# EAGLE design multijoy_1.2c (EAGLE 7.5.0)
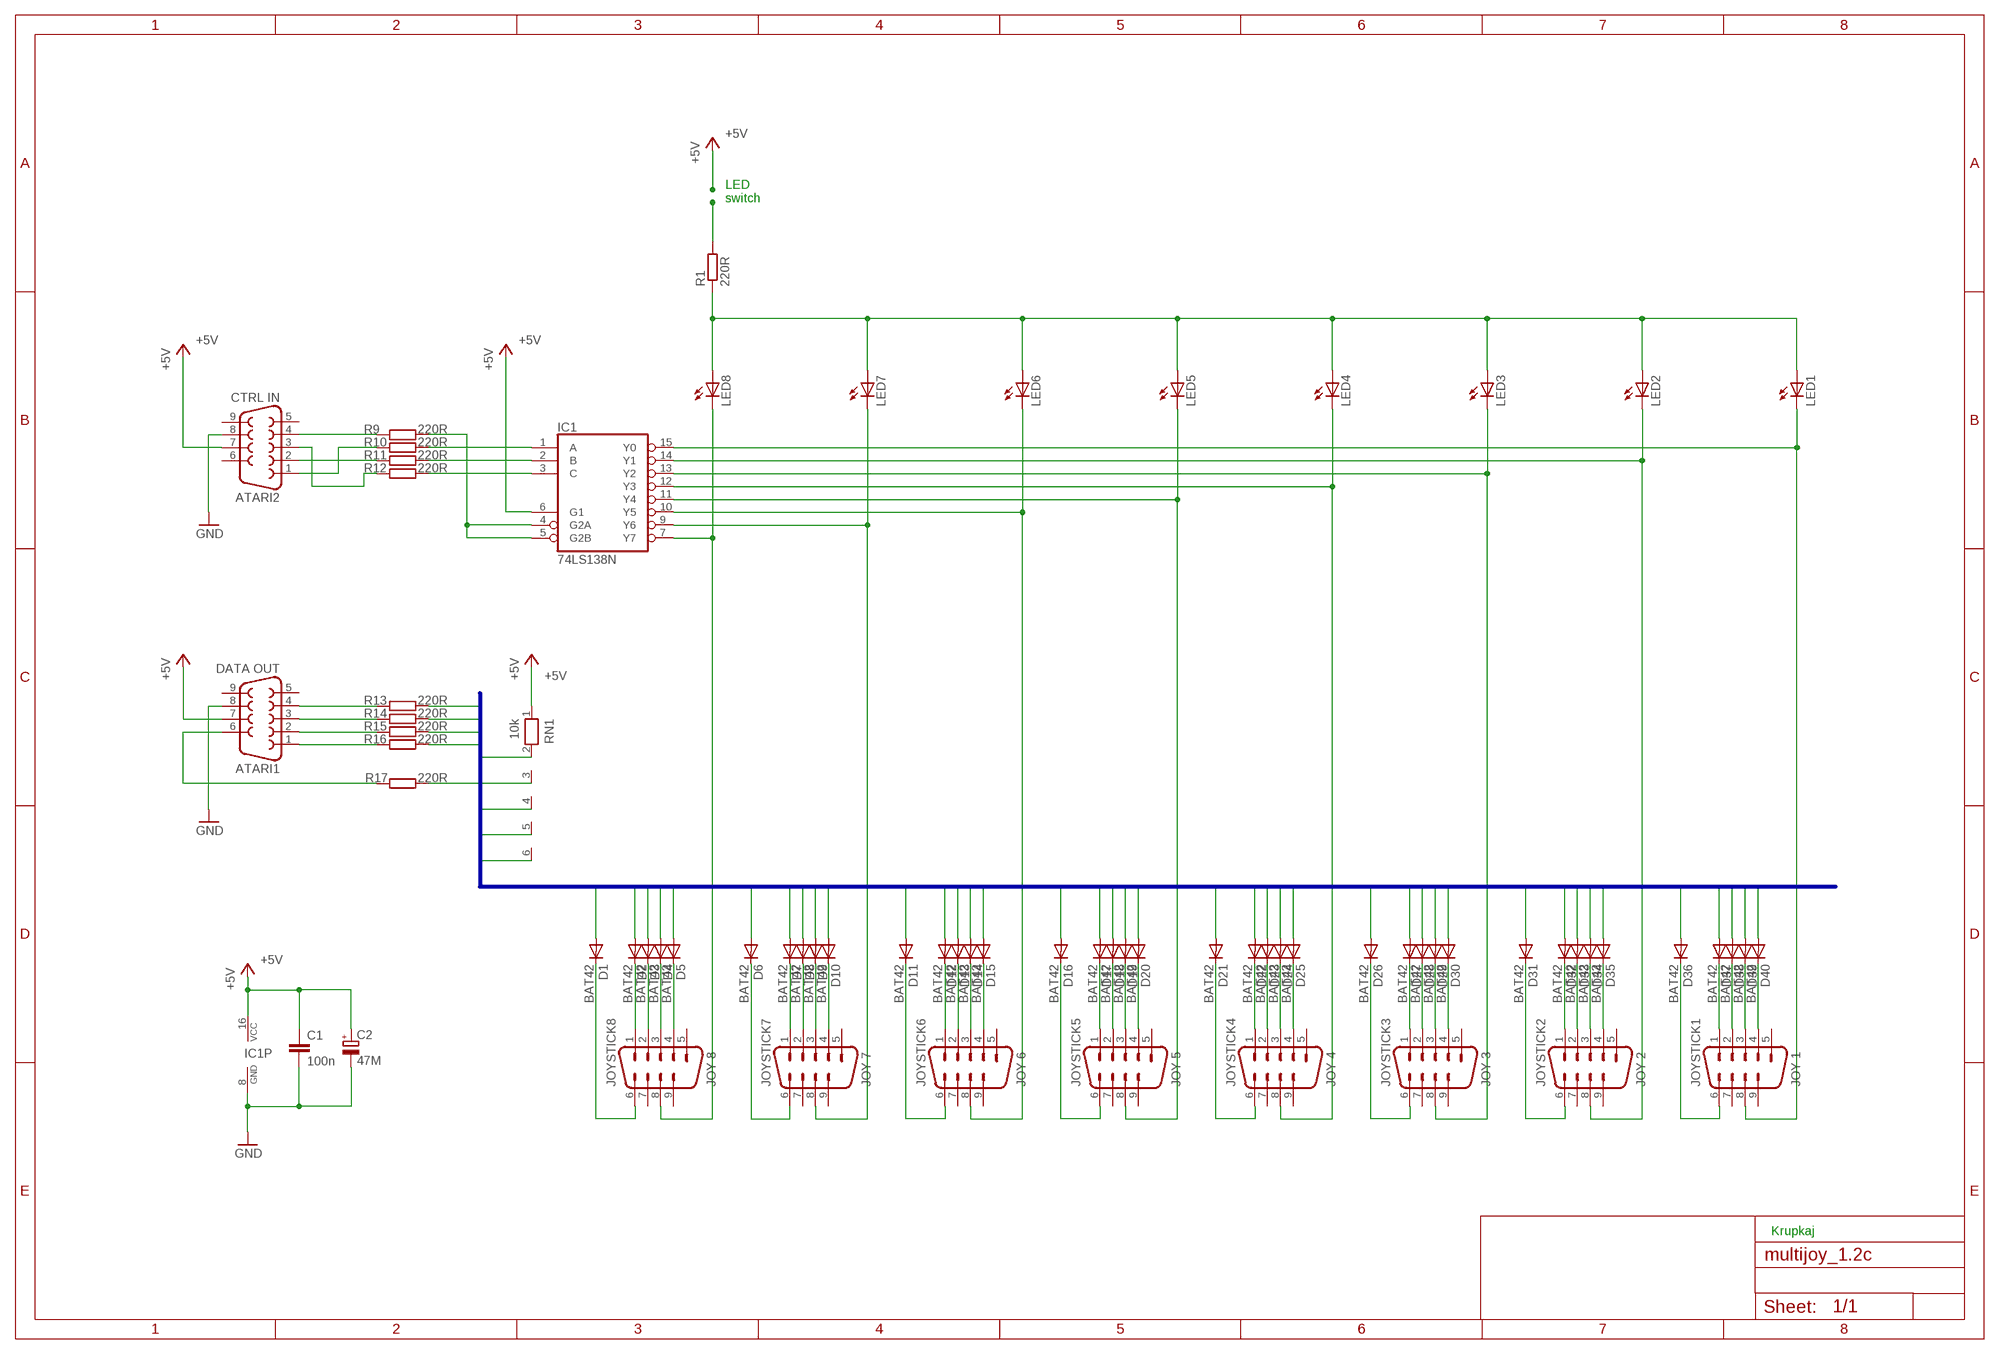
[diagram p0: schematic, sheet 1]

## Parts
ATARI1  DATA OUT  F09HP  [F09HP]
ATARI2  CTRL IN  F09HP  [F09HP]
C1  100n  C-EU050-025X075  [C050-025X075]
C2  47M  CPOL-EUE2,5-6E  [E2,5-6E]
D1  BAT42  DIODE-D-5  [D-5]
D2  BAT42  1N4148D-5  [D-5]
D3  BAT42  DIODE-D-7.5  [D-7.5]
D4  BAT42  DIODE-D-10  [D-10]
D5  BAT42  1N4148D-12.5  [D-12.5]
D6  BAT42  1N4148D-7.5  [D-7.5]
D7  BAT42  1N4148D-5  [D-5]
D8  BAT42  DIODE-D-10  [D-10]
D9  BAT42  DIODE-D-10  [D-10]
D10  BAT42  1N4148D-12.5  [D-12.5]
D11  BAT42  1N4148D-7.5  [D-7.5]
D12  BAT42  1N4148D-5  [D-5]
D13  BAT42  1N4148D-10  [D-10]
D14  BAT42  1N4148D-10  [D-10]
D15  BAT42  1N4148D-12.5  [D-12.5]
D16  BAT42  1N4148D-5  [D-5]
D17  BAT42  1N4148D-7.5  [D-7.5]
D18  BAT42  1N4148D-7.5  [D-7.5]
D19  BAT42  1N4148D-10  [D-10]
D20  BAT42  1N4148D-12.5  [D-12.5]
D21  BAT42  1N4148D-7.5  [D-7.5]
D22  BAT42  1N4148D-5  [D-5]
D23  BAT42  1N4148D-7.5  [D-7.5]
D24  BAT42  1N4148D-10  [D-10]
D25  BAT42  1N4148D-12.5  [D-12.5]
D26  BAT42  1N4148D-7.5  [D-7.5]
D27  BAT42  1N4148D-7.5  [D-7.5]
D28  BAT42  1N4148D-10  [D-10]
D29  BAT42  1N4148D-10  [D-10]
D30  BAT42  1N4148D-12.5  [D-12.5]
D31  BAT42  1N4148D-7.5  [D-7.5]
D32  BAT42  1N4148D-5  [D-5]
D33  BAT42  1N4148D-10  [D-10]
D34  BAT42  1N4148D-10  [D-10]
D35  BAT42  1N4148D-12.5  [D-12.5]
D36  BAT42  1N4148D-7.5  [D-7.5]
D37  BAT42  1N4148D-7.5  [D-7.5]
D38  BAT42  1N4148D-7.5  [D-7.5]
D39  BAT42  1N4148D-7.5  [D-7.5]
D40  BAT42  1N4148D-7.5  [D-7.5]
IC1  74LS138N  [DIL16]
JOYSTICK1  JOY 1  M09HP  [M09HP]
JOYSTICK2  JOY 2  M09HP  [M09HP]
JOYSTICK3  JOY 3  M09HP  [M09HP]
JOYSTICK4  JOY 4  M09HP  [M09HP]
JOYSTICK5  JOY 5  M09HP  [M09HP]
JOYSTICK6  JOY 6  M09HP  [M09HP]
JOYSTICK7  JOY 7  M09HP  [M09HP]
JOYSTICK8  JOY 8  M09HP  [M09HP]
LED1  LEDCHIPLED_0805  [CHIPLED_0805]
LED2  LEDCHIPLED_0805  [CHIPLED_0805]
LED3  LEDCHIPLED_0805  [CHIPLED_0805]
LED4  LEDCHIPLED_0805  [CHIPLED_0805]
LED5  LEDCHIPLED_0805  [CHIPLED_0805]
LED6  LEDCHIPLED_0805  [CHIPLED_0805]
LED7  LEDCHIPLED_0805  [CHIPLED_0805]
LED8  LEDCHIPLED_0805  [CHIPLED_0805]
R1  220R  R-EU_R0805  [R0805]
R9  220R  R-EU_R0805  [R0805]
R10  220R  R-EU_R0805  [R0805]
R11  220R  R-EU_R0805  [R0805]
R12  220R  R-EU_R0805  [R0805]
R13  220R  R-EU_R0805  [R0805]
R14  220R  R-EU_R0805  [R0805]
R15  220R  R-EU_R0805  [R0805]
R16  220R  R-EU_R0805  [R0805]
R17  220R  R-EU_R0805  [R0805]
RN1  10k  RN05  [RN-6]

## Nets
+5V: ATARI1.7 ATARI2.7 C1.1 C2.+ IC1.6(G1) IC1.16(VCC) RN1.1
+5VLED: R1.2
GND: ATARI1.8 ATARI2.8 C1.2 C2.- IC1.8(GND)
INPUT1: D2.A D7.A D12.A D17.A D22.A D27.A D32.A D37.A R16.2 RN1.6
INPUT2: D3.A D8.A D13.A D18.A D23.A D28.A D33.A D38.A R15.2 RN1.4
INPUT3: D4.A D9.A D14.A D19.A D24.A D29.A D34.A D39.A R14.2 RN1.3
INPUT4: D5.A D10.A D15.A D20.A D25.A D30.A D35.A D40.A R13.2 RN1.2
INPUT6: D1.A D6.A D11.A D16.A D21.A D26.A D31.A D36.A R17.2 RN1.5
N$1: D39.C JOYSTICK1.3
N$2: D40.C JOYSTICK1.4
N$3: D38.C JOYSTICK1.2
N$4: D37.C JOYSTICK1.1
N$5: D1.C JOYSTICK8.6
N$6: D2.C JOYSTICK8.1
N$7: D3.C JOYSTICK8.2
N$8: D4.C JOYSTICK8.3
N$9: D5.C JOYSTICK8.4
N$10: D6.C JOYSTICK7.6
N$11: D7.C JOYSTICK7.1
N$12: D8.C JOYSTICK7.2
N$13: D9.C JOYSTICK7.3
N$14: D10.C JOYSTICK7.4
N$15: D36.C JOYSTICK1.6
N$16: D35.C JOYSTICK2.4
N$17: D34.C JOYSTICK2.3
N$18: D33.C JOYSTICK2.2
N$19: D32.C JOYSTICK2.1
N$20: D31.C JOYSTICK2.6
N$21: D30.C JOYSTICK3.4
N$22: D27.C JOYSTICK3.1
N$23: D26.C JOYSTICK3.6
N$24: D25.C JOYSTICK4.4
N$25: D24.C JOYSTICK4.3
N$26: D23.C JOYSTICK4.2
N$27: D22.C JOYSTICK4.1
N$28: D21.C JOYSTICK4.6
N$29: D20.C JOYSTICK5.4
N$30: D19.C JOYSTICK5.3
N$31: D18.C JOYSTICK5.2
N$32: D17.C JOYSTICK5.1
N$33: D16.C JOYSTICK5.6
N$34: D15.C JOYSTICK6.4
N$35: D14.C JOYSTICK6.3
N$36: D13.C JOYSTICK6.2
N$37: D12.C JOYSTICK6.1
N$38: D11.C JOYSTICK6.6
N$39: D28.C JOYSTICK3.2
N$40: D29.C JOYSTICK3.3
N$41: IC1.7(Y7) JOYSTICK8.8 LED8.C
N$43: IC1.10(Y5) JOYSTICK6.8 LED6.C
N$44: IC1.11(Y4) JOYSTICK5.8 LED5.C
N$45: IC1.12(Y3) JOYSTICK4.8 LED4.C
N$46: IC1.13(Y2) JOYSTICK3.8 LED3.C
N$47: IC1.14(Y1) JOYSTICK2.8 LED2.C
N$48: IC1.15(Y0) JOYSTICK1.8 LED1.C
N$49: IC1.1(A) R10.2
N$51: ATARI2.3 R12.1
N$52: IC1.4(G2A) IC1.5(G2B) R9.2
N$67: LED1.A LED2.A LED3.A LED4.A LED5.A LED6.A LED7.A LED8.A R1.1
N$68: ATARI2.4 R9.1
N$69: ATARI2.1 R10.1
N$70: ATARI2.2 R11.1
N$71: IC1.3(C) R12.2
N$73: ATARI1.4 R13.1
N$74: ATARI1.3 R14.1
N$75: ATARI1.2 R15.1
N$76: ATARI1.1 R16.1
N$77: ATARI1.6 R17.1
N$724: IC1.9(Y6) JOYSTICK7.8 LED7.C
OUTPUT: IC1.2(B) R11.2
Unconnected: ATARI1.5 ATARI1.9 ATARI2.5 ATARI2.6 ATARI2.9 JOYSTICK1.5 JOYSTICK1.7 JOYSTICK1.9 JOYSTICK2.5 JOYSTICK2.7 JOYSTICK2.9 JOYSTICK3.5 JOYSTICK3.7 JOYSTICK3.9 JOYSTICK4.5 JOYSTICK4.7 JOYSTICK4.9 JOYSTICK5.5 JOYSTICK5.7 JOYSTICK5.9 JOYSTICK6.5 JOYSTICK6.7 JOYSTICK6.9 JOYSTICK7.5 JOYSTICK7.7 JOYSTICK7.9 JOYSTICK8.5 JOYSTICK8.7 JOYSTICK8.9

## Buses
INPUT[1..6]

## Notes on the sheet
- LED
  switch
- Krupkaj

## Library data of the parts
ATARI1 ATARI2 = con-subd-m:F09: SUB-D; OC_FARNELL: unknown; OC_NEWARK: unknown
C1 = rcl:C-EU: CAPACITOR, European symbol
C2 = rcl:CPOL-EU: POLARIZED CAPACITOR, European symbol
D1 D3 D4 D8 D9 = diode:DIODE-: DIODE
D2 D5-D7 D10-D40 = diode:1N4148: DIODE
IC1 = 74xx-eu:74*138: 3-line to 8-line DECODER/DEMULTIPLEXER
JOYSTICK1-JOYSTICK8 = con-subd-m:M09: SUB-D; OC_FARNELL: unknown; OC_NEWARK: unknown
LED1-LED8 = led:LED: LED
R1 R9-R17 = rcl:R-EU_: RESISTOR, European symbol
RN1 = resistor-net:RN05: RESISTOR NETWORK

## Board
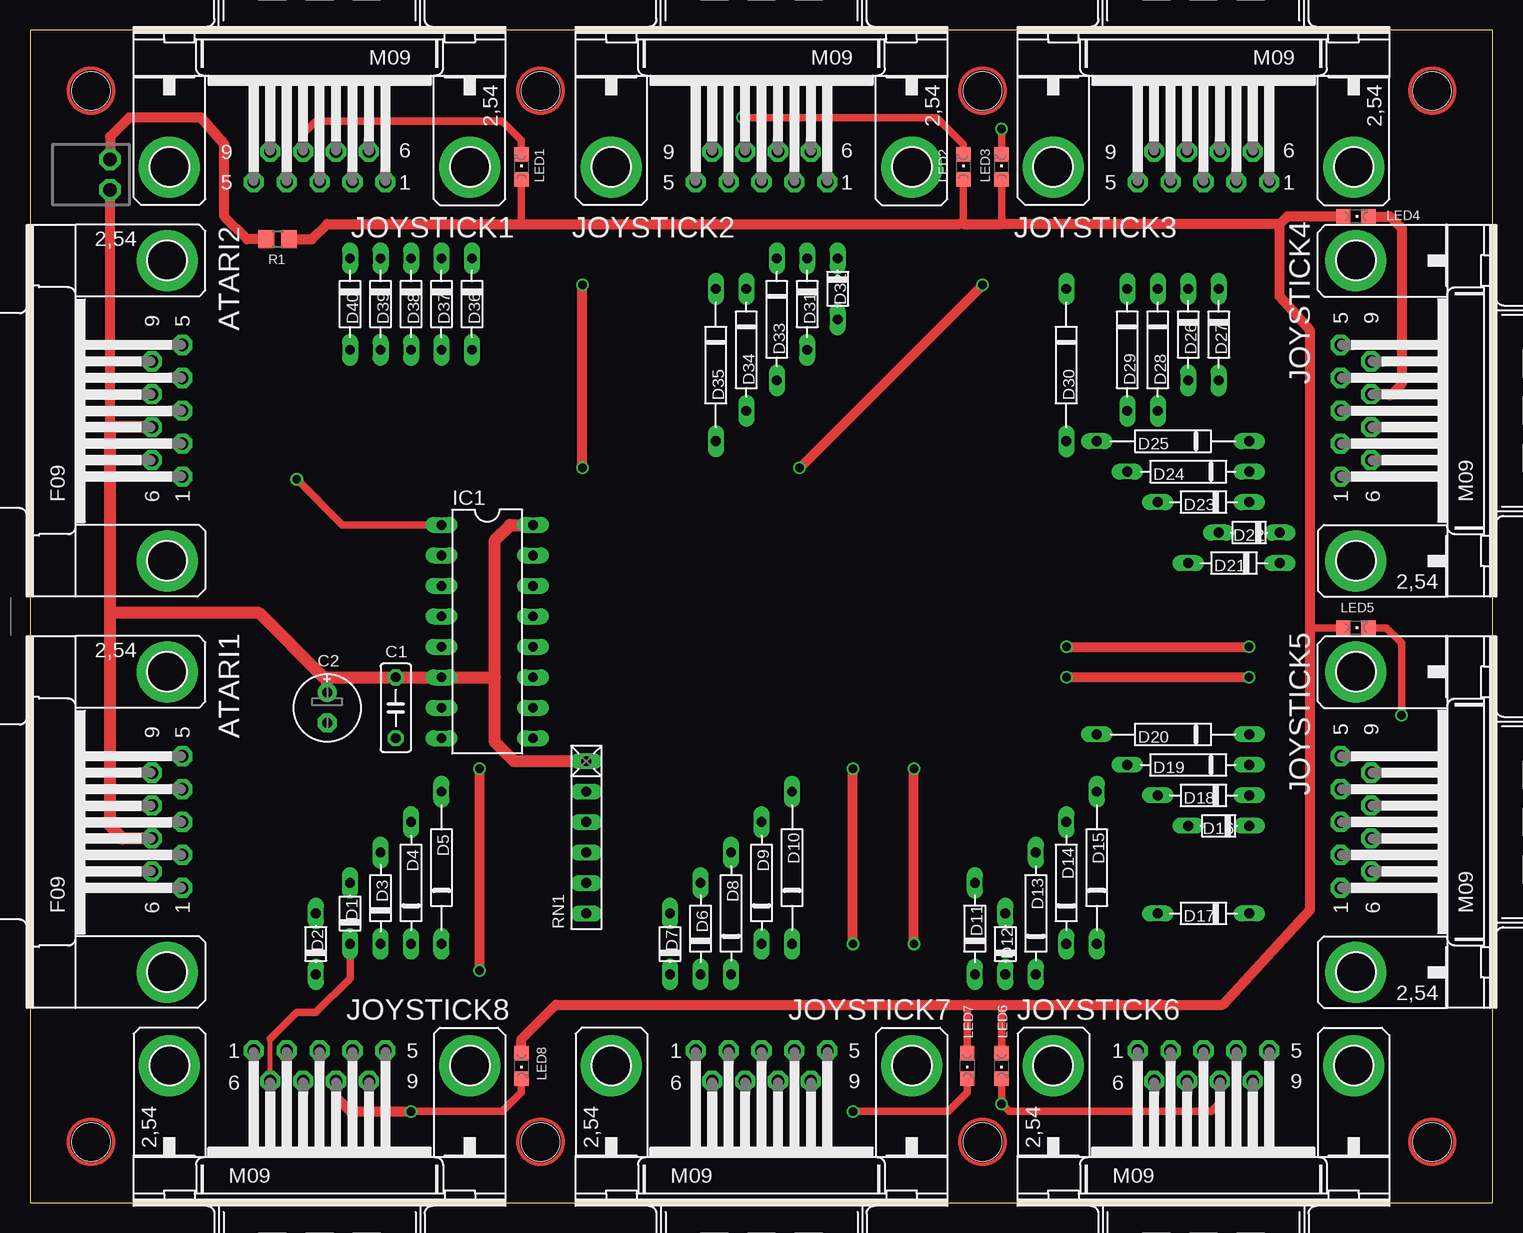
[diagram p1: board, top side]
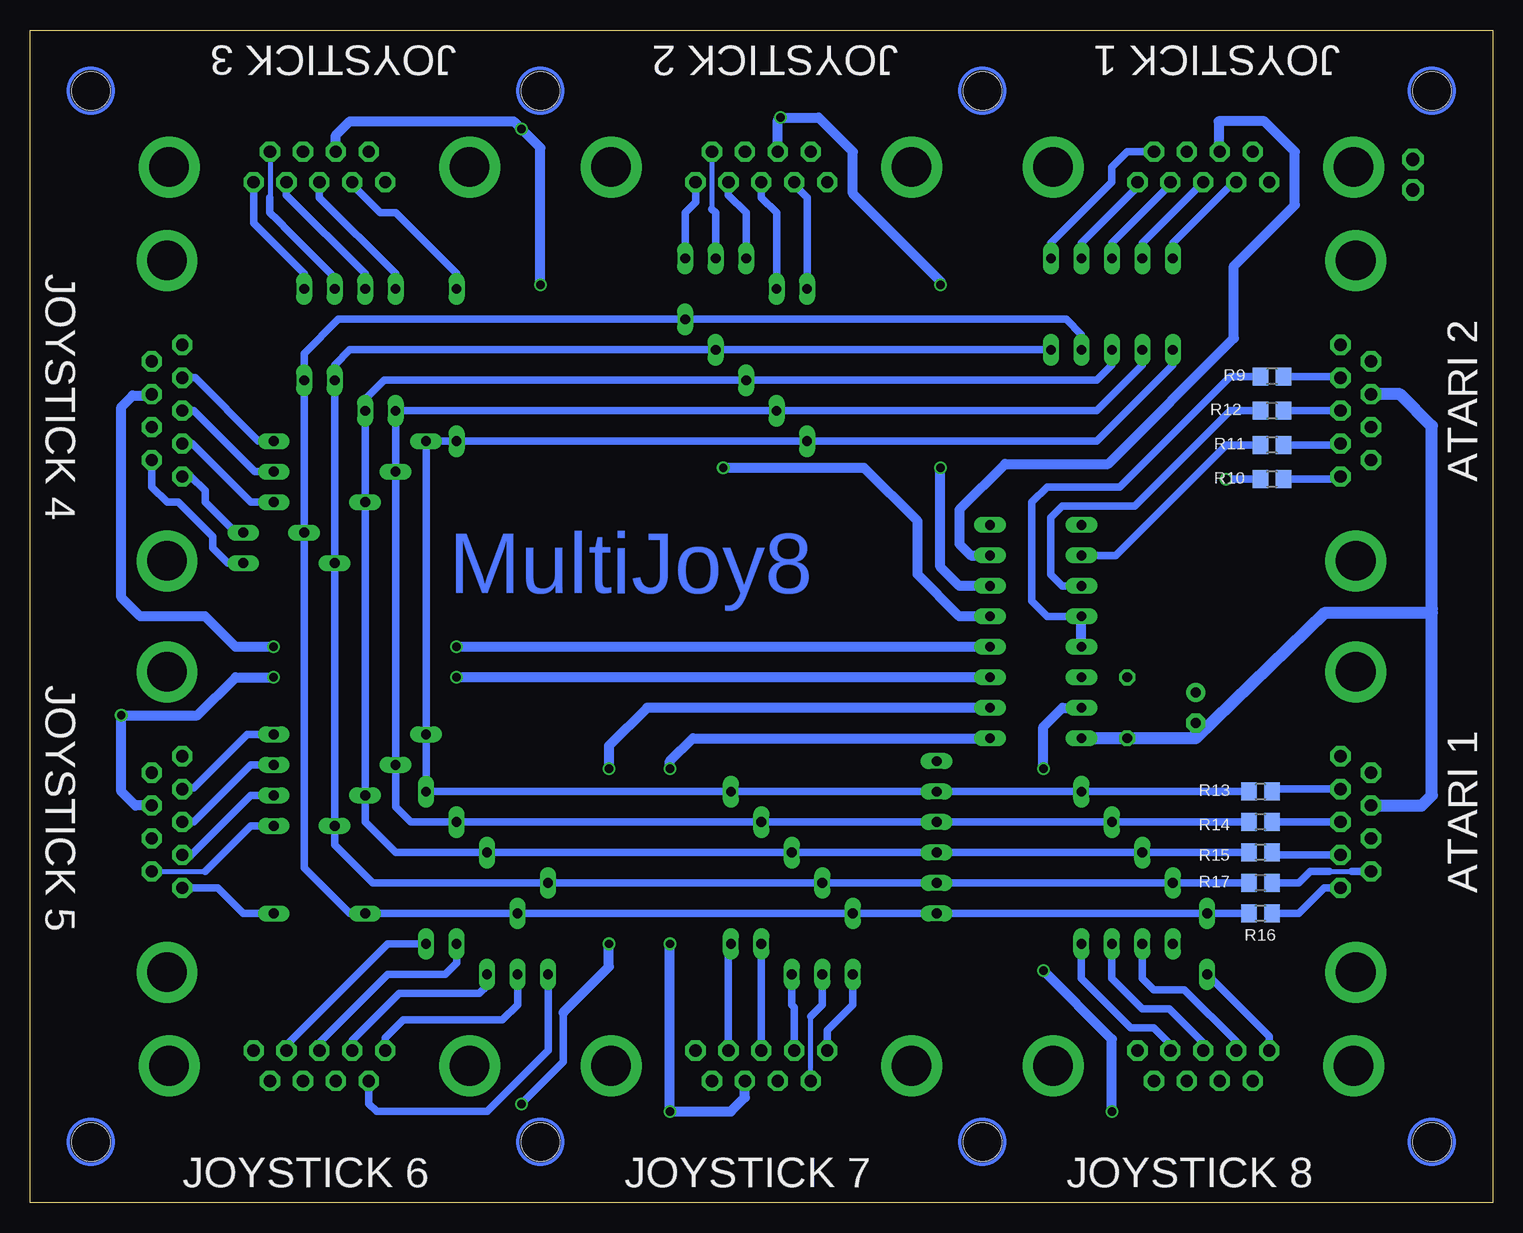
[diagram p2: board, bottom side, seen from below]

Size 121.91 x 97.78 mm. Coordinates in mm from the lower left corner, seen from the top.
Outline: 0,0 121.91,0 121.91,97.78 0,97.78 0,0
Copper layers (1*16): Top 0.035mm / dielectric 1.5mm / Bottom 0.035mm
Design rules "SeeedStudio_2layer_DRU_no_angle_20140221": minimum track width 6mil, minimum drill 12mil, track to track 6mil, track to pad 6mil, pad to pad 6mil, via to via 6mil, smd to smd 0mil, copper to edge 10mil, drill to drill 10mil, minimum pad ring 10mil, minimum via ring 6mil, stop-mask expansion 2mil, vias tented up to drill 100mil, thermal gap 10mil
Holes 3.2 mm at 5.08,92.71 42.55,92.71 79.38,92.71 116.84,92.71 116.84,5.08 79.38,5.08 42.55,5.08 5.08,5.08

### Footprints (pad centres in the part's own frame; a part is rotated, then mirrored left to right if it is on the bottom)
F09HP = drill 1.016 pad 1.676 octagon: 1 -5.486,-1.27; 2 -2.743,-1.27; 3 0,-1.27; 4 2.743,-1.27; 5 5.486,-1.27; 6 -4.115,1.27; 7 -1.372,1.27; 8 1.372,1.27; 9 4.115,1.27 | drill 3.302 pad 5.08: G1 -12.522,0; G2 12.522,0
C050-025X075 = drill 0.813 octagon: 1 -2.54,0; 2 2.54,0
E2,5-6E = drill 0.813 pad 1.575: + -1.27,0 | drill 0.813 pad 1.575 octagon: - 1.27,0
D-5 = drill 0.813 long: A 2.54,0; C -2.54,0
D-7.5 = drill 0.813 long: A 3.81,0; C -3.81,0
D-10 = drill 0.813 long: A 5.08,0; C -5.08,0
D-12.5 = drill 0.813 long: A 6.35,0; C -6.35,0
DIL16 = drill 0.813 long: 1 -8.89,-3.81; 2 -6.35,-3.81; 3 -3.81,-3.81; 4 -1.27,-3.81; 5 1.27,-3.81; 6 3.81,-3.81; 7 6.35,-3.81; 8 8.89,-3.81; 9 8.89,3.81; 10 6.35,3.81; 11 3.81,3.81; 12 1.27,3.81; 13 -1.27,3.81; 14 -3.81,3.81; 15 -6.35,3.81; 16 -8.89,3.81
M09HP = drill 1.016 pad 1.676 octagon: 1 -5.486,1.27; 2 -2.743,1.27; 3 0,1.27; 4 2.743,1.27; 5 5.486,1.27; 6 -4.115,-1.27; 7 -1.372,-1.27; 8 1.372,-1.27; 9 4.115,-1.27 | drill 3.302 pad 5.08: G1 -12.522,0; G2 12.522,0
CHIPLED_0805 = smd 1.2 x 1.2: A 0,-1.05; C 0,1.05
R0805 = smd 1.3 x 1.5: 1 -0.95,0; 2 0.95,0
RN-6 = drill 0.813 long: 1 -6.35,0; 2 -3.81,0; 3 -1.27,0; 4 1.27,0; 5 3.81,0; 6 6.35,0

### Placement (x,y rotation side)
ATARI1  11.43,31.75 90 top
ATARI2  11.43,66.04 90 top
C1  30.48,41.27 270 top
C2  24.77,41.27 270 top
D1  26.67,24.13 90 top
D2  23.81,21.59 90 top
D3  29.21,25.4 90 top
D4  31.75,26.67 90 top
D5  34.29,27.94 90 top
D6  55.88,22.86 90 top
D7  53.34,21.59 90 top
D8  58.42,24.13 90 top
D9  60.96,26.67 90 top
D10  63.5,27.94 90 top
D11  78.74,22.86 90 top
D12  81.28,21.59 90 top
D13  83.82,24.13 90 top
D14  86.36,26.67 90 top
D15  88.9,27.94 90 top
D16  99.06,31.43 180 top
D17  97.79,24.13 180 top
D18  97.79,33.97 180 top
D19  96.52,36.51 180 top
D20  95.25,39.05 180 top
D21  100.33,53.34 180 top
D22  101.6,55.88 180 top
D23  97.79,58.42 180 top
D24  96.52,60.96 180 top
D25  95.25,63.5 180 top
D26  96.52,72.39 270 top
D27  99.06,72.39 270 top
D28  93.98,71.12 270 top
D29  91.44,71.12 270 top
D30  86.36,69.85 270 top
D31  64.77,74.93 270 top
D32  67.31,76.2 270 top
D33  62.23,73.66 270 top
D34  59.69,71.12 270 top
D35  57.15,69.85 270 top
D36  36.83,74.93 270 top
D37  34.29,74.93 270 top
D38  31.75,74.93 270 top
D39  29.21,74.93 270 top
D40  26.67,74.93 270 top
IC1  38.1,47.62 270 top
JOYSTICK1  24.13,86.36 180 top
JOYSTICK2  60.96,86.36 180 top
JOYSTICK3  97.79,86.36 180 top
JOYSTICK4  110.49,66.04 90 top
JOYSTICK5  110.49,31.75 90 top
JOYSTICK6  97.79,11.43 0 top
JOYSTICK7  60.96,11.43 0 top
JOYSTICK8  24.13,11.43 0 top
LED1  40.96,86.36 0 top
LED2  77.79,86.36 0 top
LED3  80.96,86.36 0 top
LED4  110.49,82.23 270 top
LED5  110.49,47.94 270 top
LED6  80.96,11.43 180 top
LED7  78.1,11.43 180 top
LED8  40.96,11.43 180 top
R1  20.64,80.33 180 top
R9  18.41,68.9 180 bottom
R10  18.41,60.33 180 bottom
R11  18.41,63.18 180 bottom
R12  18.41,66.04 180 bottom
R13  19.37,34.29 180 bottom
R14  19.37,31.75 180 bottom
R15  19.37,29.21 180 bottom
R16  19.37,24.13 180 bottom
R17  19.37,26.67 180 bottom
RN1  46.36,30.48 270 top

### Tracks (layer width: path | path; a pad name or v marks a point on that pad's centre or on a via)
+5V  (via drill 1.1 pad 1.78)
  Top 0.813: 6.67,64.67 v6.67,84.45 | 6.67,31.75 6.67,31.43
  Top 1.016: IC1.16 40,56.52 38.73,55.25 38.73,43.81 | 38.73,43.81 IC1.6 C1.1 24.77,43.81 | 6.67,49.21 19.05,49.21 24.45,43.81 24.77,43.81 | 38.73,43.81 38.73,38.42 40.32,36.83 RN1.1 | C2.+ 24.77,43.81 | ATARI2.7 6.67,64.67 6.67,49.21 | ATARI1.7 7.72,30.38 6.67,31.43 | 6.67,31.75 6.67,49.21
+5VLED  (via drill 1.1 pad 1.78)
  Top 0.813: R1.2 18.1,80.33 16.19,82.23 16.19,88.27 14.29,90.49 8.26,90.49 6.67,88.9 v6.67,86.99
GND
  Bottom 1.016: 24.77,38.73 13.97,49.21 5.08,49.21 | 5.08,49.21 5.08,49.53 5.08,64.77 7.72,67.41 ATARI2.8 | 24.77,38.73 C1.2 IC1.8 | C2.- 24.77,38.73 | ATARI1.8 5.93,33.12 5.08,33.97 5.08,49.21
INPUT1
  Bottom 0.61: D37.A 34.29,72.39 35.56,73.66 D32.A 96.2,73.66 99.06,70.8 D27.A D22.A 99.06,27.94 95.25,24.13 D17.A D12.A D7.A RN1.6 D2.A R16.2
INPUT2
  Bottom 0.61: D38.A 31.75,69.85 33.02,68.58 D33.A 92.39,68.58 93.98,66.99 D28.A D23.A D18.A 93.98,31.75 91.44,29.21 D13.A D8.A RN1.4 D3.A R15.2
INPUT3
  Bottom 0.61: D39.A 29.21,69.85 33.02,66.04 D34.A D29.A D24.A D19.A 91.44,33.02 90.17,31.75 D14.A D9.A RN1.3 D4.A R14.2
INPUT4
  Bottom 0.61: D40.A 26.67,69.85 33.02,63.5 D35.A D30.A D25.A D20.A D15.A D10.A RN1.2 D5.A R13.2
INPUT6
  Bottom 0.61: D36.A D31.A 95.25,71.12 96.52,69.85 D26.A D21.A D16.A 96.52,29.84 93.34,26.67 D11.A D6.A RN1.5 D1.A R17.2
N$1
  Bottom 0.406: 29.21,80.01 D39.C
  Bottom 0.61: JOYSTICK1.3 29.21,80.01
N$2
  Bottom 0.406: JOYSTICK1.4 21.39,85.29 | 26.67,80.01 D40.C
  Bottom 0.61: 21.39,85.29 26.67,80.01
N$3
  Bottom 0.406: JOYSTICK1.2 26.87,84.89 | 31.75,80.01 D38.C
  Bottom 0.61: 26.87,84.89 31.75,80.01
N$4
  Bottom 0.406: JOYSTICK1.1 29.62,84.68 | 34.29,80.01 D37.C
  Bottom 0.61: 29.62,84.68 34.29,80.01
N$5
  Top 0.406: JOYSTICK8.6 20.02,13.66
  Top 0.61: 20.02,13.66 22.23,15.88 23.81,15.88 26.67,18.73 D1.C
N$6
  Bottom 0.61: JOYSTICK8.1 18.64,13.88 D2.C
N$7
  Bottom 0.61: JOYSTICK8.2 21.39,13.45 25.72,17.78 28.26,17.78 29.21,18.73 D3.C
N$8
  Bottom 0.61: JOYSTICK8.3 24.13,13.34 26.99,16.19 29.21,16.19 31.75,18.73 D4.C
N$9
  Bottom 0.61: JOYSTICK8.4 26.87,13.22 28.26,14.61 30.16,14.61 34.29,18.73 D5.C
N$10
  Bottom 0.406: JOYSTICK7.6 56.84,15.54
  Bottom 0.61: 56.84,15.54 55.88,16.51 D6.C
N$11
  Bottom 0.61: JOYSTICK7.1 55.47,14.38 53.34,16.51 D7.C
N$12
  Bottom 0.61: JOYSTICK7.2 58.22,16.31 58.42,16.51 D8.C
N$13
  Bottom 0.61: D9.C JOYSTICK7.3
N$14
  Bottom 0.61: JOYSTICK7.4 63.7,21.39 D10.C
N$15
  Bottom 0.406: 36.83,80.01 D36.C
  Bottom 0.61: JOYSTICK1.6 30.48,87.63 31.75,86.36 31.75,85.09 36.83,80.01
N$16
  Bottom 0.406: JOYSTICK2.4 58.22,84.89
  Bottom 0.61: 58.22,84.89 57.15,83.82 D35.C
N$17
  Bottom 0.61: JOYSTICK2.3 60.96,83.82 59.69,82.55 D34.C
N$18
  Bottom 0.61: JOYSTICK2.2 63.7,84.02 62.23,82.55 D33.C
N$19
  Bottom 0.61: JOYSTICK2.1 66.45,83.41 67.31,82.55 D32.C
N$20
  Bottom 0.406: JOYSTICK2.6 65.08,82.85
  Bottom 0.61: 65.08,82.85 64.77,82.55 D31.C
N$21
  Bottom 0.61: D30.C 86.36,77.47 91.44,82.55 92.71,82.55 95.05,84.89 JOYSTICK3.4
N$22
  Bottom 0.61: D27.C 99.06,77.47 103.28,81.69 JOYSTICK3.1
N$23
  Bottom 0.406: JOYSTICK3.6 101.91,83.83 101.92,83.82
  Bottom 0.61: D26.C 96.52,77.15 100.33,80.96 101.28,81.91 101.92,82.55 101.92,83.82
N$24
  Bottom 0.61: JOYSTICK4.4 108.15,68.78 102.87,63.5 D25.C
N$25
  Bottom 0.61: D24.C 103.19,60.96 108.27,66.04 JOYSTICK4.3
N$26
  Bottom 0.61: D23.C 103.5,58.42 108.38,63.3 JOYSTICK4.2
N$27
  Bottom 0.61: 109.22,60.96 JOYSTICK4.1 108.5,60.55 107.31,59.37 107.31,58.42 105.09,56.2 104.77,55.88 D22.C
N$28
  Bottom 0.61: JOYSTICK4.6 111.76,59.69 110.49,58.42 109.54,58.42 106.68,55.56 106.68,54.61 105.41,53.34 D21.C
N$29
  Bottom 0.406: 109.11,34.61 JOYSTICK5.4
  Bottom 0.61: D20.C 103.82,39.05 108.27,34.61 109.11,34.61
N$30
  Bottom 0.61: D19.C 103.5,36.51 108.27,31.75 JOYSTICK5.3
N$31
  Bottom 0.406: 109.11,28.89 JOYSTICK5.2
  Bottom 0.61: D18.C 103.5,33.97 108.58,28.89 109.11,28.89
N$32
  Bottom 0.61: D17.C 104.14,24.13 106.27,26.26 JOYSTICK5.1
N$33
  Bottom 0.406: JOYSTICK5.6 107.3,27.64
  Bottom 0.61: 107.3,27.64 103.5,31.43 D16.C
N$34
  Bottom 0.61: D15.C 92.08,21.59 100.53,13.13 JOYSTICK6.4
N$35
  Bottom 0.61: JOYSTICK6.3 97.79,13.34 92.08,19.05 87.31,19.05 86.36,20 D14.C
N$36
  Bottom 0.61: JOYSTICK6.2 95.05,13.54 91.12,17.46 84.45,17.46 83.82,18.1 D13.C
N$37
  Bottom 0.61: D12.C 81.28,16.51 82.55,15.24 90.8,15.24 92.3,13.74 JOYSTICK6.1
N$38
  Bottom 0.61: JOYSTICK6.6 93.66,8.26 93.03,7.62 83.82,7.62 78.74,12.7 D11.C
N$39
  Bottom 0.61: JOYSTICK3.2 100.53,84.02 93.98,77.47 D28.C
N$40
  Bottom 0.61: D29.C 91.44,77.47 97.79,83.82 JOYSTICK3.3
N$41  (via drill 0.7)
  Top 0.61: LED8.C 40.96,9.21 39.37,7.62 v31.75,7.62
  Top 0.813: v37.47,19.37 v37.47,36.2 | JOYSTICK8.8 25.5,8.79 26.67,7.62 v31.75,7.62
  Bottom 0.813: v31.75,7.62 31.75,13.65 v37.47,19.37 | v37.47,36.2 37.47,39.69 35.88,41.27 IC1.7
N$43  (via drill 0.7)
  Top 0.61: LED6.C v80.96,8.26 81.6,7.62 98.42,7.62 99.16,8.36 JOYSTICK6.8
  Top 0.813: v73.66,21.59 v73.66,36.2
  Bottom 0.61: 77.47,15.88 77.47,11.75 v80.96,8.26
  Bottom 0.813: v73.66,36.2 73.66,38.1 70.48,41.27 IC1.10 | 77.47,15.88 73.66,19.69 v73.66,21.59
N$44  (via drill 0.7)
  Top 0.61: v114.3,40.64 114.3,46.67 113.03,47.94 LED5.C
  Top 0.813: v101.6,43.81 v86.36,43.81
  Bottom 0.813: IC1.11 v86.36,43.81 | v101.6,43.81 104.77,43.81 107.95,40.64 v114.3,40.64 114.3,34.29 113.13,33.12 JOYSTICK5.8
N$45  (via drill 0.7)
  Top 0.813: v86.36,46.36 v101.6,46.36 | LED4.C 113.35,82.23 114.3,81.28 114.3,68.26 113.35,67.31 113.25,67.41 JOYSTICK4.8
  Bottom 0.406: 111.86,67.31 JOYSTICK4.8
  Bottom 0.813: IC1.12 v86.36,46.36 | v101.6,46.36 104.77,46.36 107.31,48.89 112.71,48.89 114.3,50.48 114.3,66.36 113.35,67.31 111.86,67.31
N$46  (via drill 0.7)
  Top 0.61: v80.96,89.53 LED3.C
  Top 0.813: v64.14,61.28 v79.38,76.52
  Bottom 0.813: IC1.13 44.45,48.89 47.94,52.39 47.94,56.83 52.39,61.28 v64.14,61.28 | v79.38,76.52 79.38,87.95 v80.96,89.53 81.6,90.17 95.25,90.17 96.42,89 JOYSTICK3.8
N$47  (via drill 0.7)
  Top 0.61: LED2.C 77.79,88.27 75.56,90.49 v59.37,90.49
  Top 0.813: v46.04,61.28 v46.04,76.52
  Bottom 0.406: 59.59,90.27 v59.37,90.49
  Bottom 0.813: IC1.14 44.45,51.44 46.04,53.02 v46.04,61.28 | v59.37,90.49 56.2,90.49 53.34,87.63 53.34,84.14 46.04,76.83 v46.04,76.52 | JOYSTICK2.8 59.59,90.27
N$48
  Top 0.61: LED1.C 40.96,88.58 39.37,90.17 23.81,90.17 22.76,89.12 JOYSTICK1.8
  Bottom 0.406: JOYSTICK1.8 22.86,87.63
  Bottom 0.813: 22.86,87.63 22.86,90.17 19.05,90.17 16.51,87.63 16.51,83.19 21.59,78.1 21.59,72.07 32.07,61.59 40.64,61.59 44.45,57.78 44.45,54.93 43.5,53.97 IC1.15
N$49  (via drill 0.7)
  Top 0.61: IC1.1 26.04,56.52 v22.23,60.33
  Bottom 0.61: v22.23,60.33 R10.2
N$51
  Bottom 0.61: R12.1 ATARI2.3
N$52
  Bottom 0.61: R9.2 21.91,68.9 31.11,59.69 37.15,59.69 38.42,58.42 38.42,50.17 37.15,48.89 IC1.4
  Bottom 0.813: IC1.5 IC1.4
N$67
  Top 0.406: 77.79,81.6 77.79,81.91 77.47,81.6
  Top 0.61: LED6.A 80.96,16.51 | LED7.A 78.1,16.51 | 106.68,47.94 LED5.A | 80.96,81.6 LED3.A | LED2.A 77.79,81.91 | LED1.A 40.96,81.6
  Top 0.813: LED8.A 40.96,13.65 43.81,16.51 78.1,16.51 80.96,16.51 99.38,16.51 106.68,24.45 106.68,47.94 106.68,72.71 104.14,75.56 104.14,81.6 | 104.14,81.6 80.96,81.6 77.79,81.6 | 77.47,81.6 40.96,81.6 24.77,81.6 23.49,80.33 R1.1 | LED4.A 104.77,82.23 104.14,81.6
N$68
  Bottom 0.406: 12.81,68.9 ATARI2.4
  Bottom 0.61: R9.1 12.81,68.9
N$69
  Bottom 0.406: 12.93,60.33 ATARI2.1
  Bottom 0.61: R10.1 12.93,60.33
N$70
  Bottom 0.406: 12.81,63.18 ATARI2.2
  Bottom 0.61: R11.1 12.81,63.18
N$71
  Bottom 0.61: R12.2 21.91,66.04 29.84,58.1 35.88,58.1 36.83,57.15 36.83,52.39 35.88,51.44 IC1.3
N$73
  Bottom 0.406: 18.21,34.49 R13.1
  Bottom 0.61: ATARI1.4 18.21,34.49
N$74
  Bottom 0.61: ATARI1.3 R14.1
N$75
  Bottom 0.406: 18.21,29.01 R15.1
  Bottom 0.61: ATARI1.2 18.21,29.01
N$76
  Bottom 0.61: ATARI1.1 14.06,26.26 16.19,24.13 R16.1
N$77
  Bottom 0.406: 13.65,27.62 11.75,27.62
  Bottom 0.61: R17.1 16.19,26.67 15.23,27.64 13.98,27.64 13.65,27.62 | 11.75,27.62 10.17,27.62 ATARI1.6
N$724  (via drill 0.7)
  Top 0.61: v68.58,7.62 76.52,7.62 78.1,9.21 LED7.C
  Top 0.813: v68.58,21.59 v68.58,36.2
  Bottom 0.813: v68.58,21.59 v68.58,7.62 63.5,7.62 62.33,8.79 JOYSTICK7.8 | v68.58,36.2 68.58,36.83 66.67,38.73 IC1.9
OUTPUT
  Bottom 0.61: R11.2 22.23,63.18 31.43,53.97 IC1.2
(copper drawn outside any net)
  shapes: Bottom circle x8, Top circle x8

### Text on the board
Bottom: MultiJoy8
bNames: JOYSTICK 1 | JOYSTICK 2 | JOYSTICK 3 | JOYSTICK 4 | ATARI 2 | JOYSTICK 5 | ATARI 1 | JOYSTICK 8 | JOYSTICK 7 | JOYSTICK 6
Document: JOYSTICK 1 | JOYSTICK 2 | JOYSTICK 3 | JOYSTICK 4 | ATARI 2 | MultiJoy8 | JOYSTICK 5 | ATARI 1 | JOYSTICK 8 | JOYSTICK 7 | JOYSTICK 6
tDocu: LED | MultiJoy8 | Original Design 1998 / Raster/ZdenekB/Musil | PCB v1.2C / krupkaj / 2019 | Olomouc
